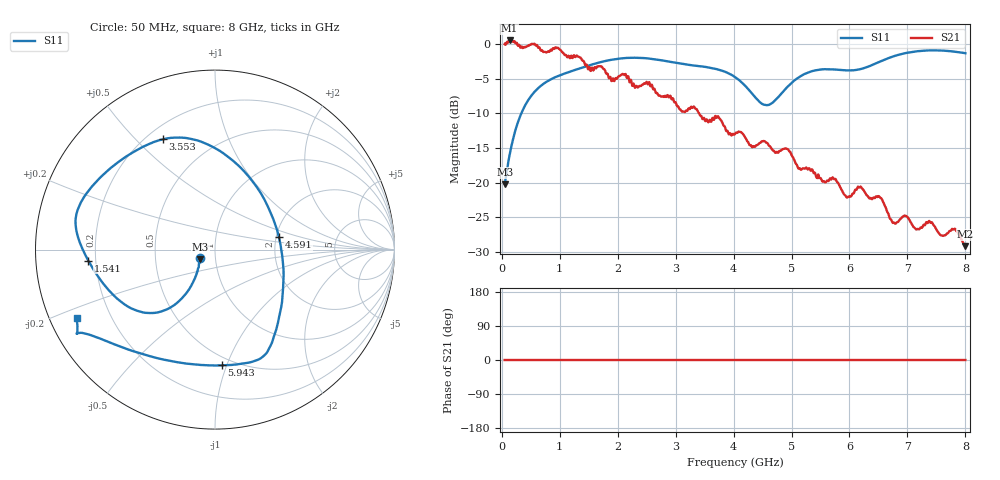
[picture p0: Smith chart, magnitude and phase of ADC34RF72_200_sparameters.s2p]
! Texas Instruments, Inc.
! ADC34RF72 - Single Channel S-Parameters - Fs = 1.5 GSPS, Termination = 200
! Port 1 represents the 200-ohm differential input, Port 2 represents the digital output of the ADC
! freq  magS11  angS11  magS21  angS21  magS12  angS12  magS22  angS22
# Hz S ma R 200
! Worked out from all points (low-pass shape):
!   1601 points, 50 MHz to 8 GHz, reference 200 ohm
!   highest |S21| = 0.52 dB at 134.5 MHz (marker M1); lowest = -29.2 dB at 8 GHz (marker M2)
!   |S21| within 3 dB of the highest: start of sweep to 1.415 GHz
!   lowest |S11| = -20.2 dB at 54.97 MHz (marker M3), VSWR 1.22, Z = 169 - j18.3 ohm
!   |S11| at or under -10 dB: start of sweep to 339.5 MHz
!   S12 and S22 are empty: the file has one direction only
!   S11 on the Smith chart (normalised r, x): 50 MHz: 0.84, -0.08; 1.541 GHz: 0.17, -0.04; 3.553 GHz: 0.26, +0.60; 4.591 GHz: 2.07, +0.33; 5.943 GHz: 0.43, -0.96; 8 GHz: 0.08, -0.23
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5e7  0.09824 -150.2  1 0.0  0 0.0  0 0.0
5.496875e7  0.09725 -146.5  1.01 0.0  0 0.0  0 0.0
1.344688e8  0.1576 -129.3  1.062 0.0  0 0.0  0 0.0
3.034062e8  0.2901 -123.4  0.9858 0.0  0 0.0  0 0.0
5.319688e8  0.4348 -129.4  1.002 0.0  0 0.0  0 0.0
8.996562e8  0.5707 -145.1  0.9252 0.0  0 0.0  0 0.0
1.376656e9  0.6739 -168.2  0.7784 0.0  0 0.0  0 0.0
1.540625e9  0.7085 -175.0  0.6442 0.0  0 0.0  0 0.0
2.151781e9  0.7941 168.1  0.5825 0.0  0 0.0  0 0.0
2.703312e9  0.7705 152.8  0.427 0.0  0 0.0  0 0.0
3.552969e9  0.68 115.4  0.2762 0.0  0 0.0  0 0.0
4.025e9  0.5775 92.2  0.2246 0.0  0 0.0  0 0.0
4.293312e9  0.4523 66.3  0.1863 0.0  0 0.0  0 0.0
4.591438e9  0.3627 10.8  0.1908 0.0  0 0.0  0 0.0
4.979e9  0.5142 -45.8  0.1661 0.0  0 0.0  0 0.0
5.351656e9  0.6372 -62.5  0.1246 0.0  0 0.0  0 0.0
5.942938e9  0.646 -86.7  0.07888 0.0  0 0.0  0 0.0
6.186406e9  0.6591 -107.0  0.09344 0.0  0 0.0  0 0.0
6.678312e9  0.7933 -140.2  0.05815 0.0  0 0.0  0 0.0
7.135438e9  0.8849 -148.4  0.04647 0.0  0 0.0  0 0.0
7.806219e9  0.8823 -150.3  0.04606 0.0  0 0.0  0 0.0
8e9  0.8594 -153.7  0.03472 0.0  0 0.0  0 0.0
